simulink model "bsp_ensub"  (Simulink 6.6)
settings: Solver=VariableStepDiscrete  SolverMode=SingleTasking  StartTime=0.0  StopTime=10.0  FixedStep=0.01  RelTol=1e-3

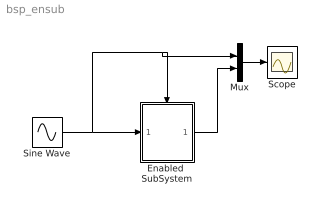
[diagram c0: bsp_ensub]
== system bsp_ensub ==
  Enabled  SubSystem : Subsystem
  Mux : Mux  Inputs=2
  Scope : Scope
  Sine Wave : Sin  SampleTime=0
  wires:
  Sine Wave/1 -> Enabled  SubSystem/1(In1), Mux/1, Enabled  SubSystem/Enable
  Mux/1 -> Scope/1
  Enabled  SubSystem/1(Out1) -> Mux/2

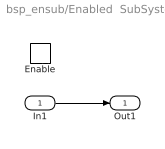
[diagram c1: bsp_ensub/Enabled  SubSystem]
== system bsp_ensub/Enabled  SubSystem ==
  In1 : Inport
  Enable : EnablePort
  Out1 : Outport
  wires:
  In1/1 -> Out1/1
